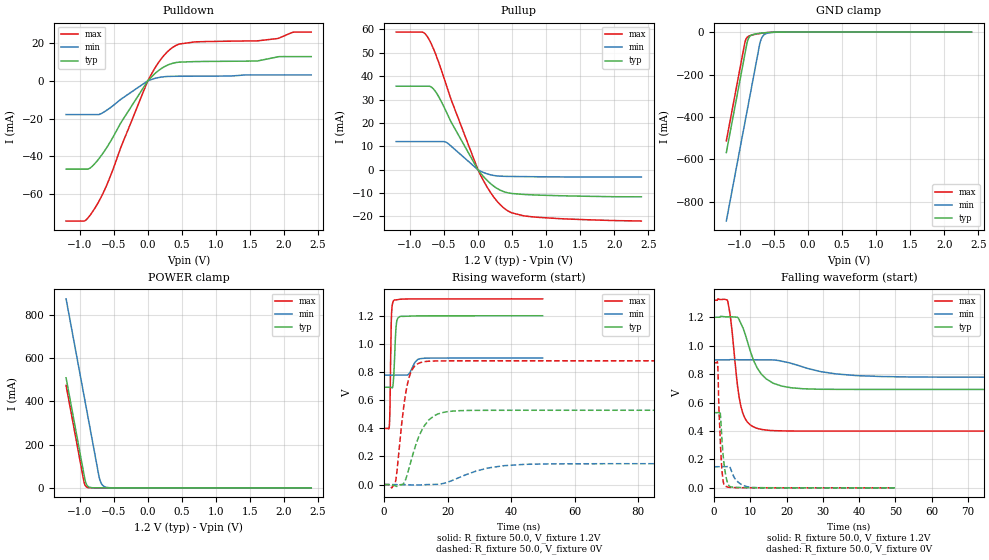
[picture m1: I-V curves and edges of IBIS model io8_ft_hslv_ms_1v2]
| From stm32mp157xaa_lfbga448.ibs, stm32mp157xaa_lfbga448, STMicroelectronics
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[Model]   io8_ft_hslv_ms_1v2
Model_type I/O
Polarity   Non-Inverting
Enable   Active-Low
| CAP_THRESHOLD on pad IOFT is "UDTCAPC" :
| Rising=20.00f vddiom   Falling=80.00f vddiom
| C_comp min and max val. don't necessarily correlate with the min and max pvt
| but are the smallest and greatest pad capacitance found.
| var   typ   min   max
C_comp   3.08865pF  3.06550pF  3.10825pF
|C_comp_pullup   1.81640pF  1.58310pF  1.74795pF
|C_comp_pulldown   1.27225pF  1.48240pF  1.36030pF
Vinl = 360.0mV
Vinh = 792.0mV
Vmeas = 600.0mV   | Reference voltage for timing measurements
Cref  = 50.0pF   | Timing specification test load capacitance value
Rref  = 100.0MOhm   | Timing specification test load resistance value
Vref  = 0V   | Timing specification test load voltage
[Model Spec]
| TIME_THRESHOLD on pin ZIV11 is "CMOS" :
| Rising=40.00f vdd   Falling=60.00f vdd
Vinl 463.60000mV 362.60000mV 506.60000mV
Vinh 741.40000mV 545.40000mV 817.40000mV
| variable   typ   min   max
[Temperature Range] 25.0 140.0 -40.0
| variable   typ   min   max
[Voltage Range] 1.2V 900.0mV 1.32V
| variable   typ   min   max
[POWER Clamp Reference] 1.2V 900.0mV 1.32V
| variable   typ   min   max
[GND Clamp Reference] 0V 0V 0V
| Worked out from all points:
|   slope of the pulldown table from 0 to 0.18 V, typ, clamps not added: 30 ohm
|   slope of the pullup table from 0 to 0.18 V, typ, clamps not added: 31.1 ohm
|   GND clamp passes 1 mA (typ) near -0.52 V on its own axis
|   POWER clamp passes 1 mA (typ) near -0.83 V on its own axis
|   rising waveform, R_fixture 50.0, V_fixture 1.2V: 20-80 % time 608ps typ, 1.71ns min, 359ps max; typ from 0.692 V to 1.2 V
|   falling waveform, R_fixture 50.0, V_fixture 1.2V: 20-80 % time 4.95ns typ, 12.1ns min, 2.49ns max; typ from 1.2 V to 0.692 V
|   rising waveform, R_fixture 50.0, V_fixture 0V: 20-80 % time 5.1ns typ, 11.5ns min, 2.82ns max; typ from 0 V to 0.528 V
|   falling waveform, R_fixture 50.0, V_fixture 0V: 20-80 % time 1.12ns typ, 2.37ns min, 843ps max; typ from 0.528 V to 0 V
[POWER Clamp]
-1.2V     508.8mA    874.1mA    473.5mA
-940mV    66.83mA    432.1mA    31.5mA
-930mV    49.83mA    415.1mA    19.15mA
-910mV    22.88mA    381.1mA    7.077mA
-880mV    7.117mA    330.1mA    1.59mA
-830mV    1.017mA    245.1mA    132uA
-720mV    14.05uA    58.12mA    554nA
-690mV    4.373uA    25.03mA    124.7nA
-650mV    922.4nA    8.136mA    17.22nA
-600mV    132.5nA    1.998mA    1.555nA
-490mV    2.736nA    90.9uA     103pA
2.4V      0A         0A         0A
[GND Clamp]
-1.2V     -567.2mA   -889.7mA   -512.2mA
-930mV    -108.2mA   -430.7mA   -53.23mA
-920mV    -91.21mA   -413.7mA   -40.49mA
-890mV    -43.51mA   -362.7mA   -23.59mA
-860mV    -22.57mA   -311.7mA   -17.89mA
-810mV    -12.11mA   -226.7mA   -13.23mA
-710mV    -6.053mA   -57.05mA   -7.064mA
-680mV    -4.908mA   -27.37mA   -5.632mA
-640mV    -3.605mA   -11.51mA   -3.985mA
-560mV    -1.665mA   -3.218mA   -1.61mA
-360mV    -34.72uA   -209.4uA   -9.248uA
2.4V      3.381nA    1.198uA    162.5pA
| variable   typ   min   max
[Pullup Reference] 1.2V 900.0mV 1.32V
| variable   typ   min   max
[Pulldown Reference] 0V 0V 0V
[Pullup]
-1.2V     35.71mA    12.03mA    58.89mA
-820mV    35.71mA    12.03mA    58.89mA
-730mV    35.71mA    12.03mA    56.33mA
-620mV    33.3mA     12.03mA    49.33mA
-460mV    24.5mA     11.63mA    35.82mA
-400mV    20.74mA    10.25mA    30.47mA
0V        5.9pA      1.254nA    2.839pA
200mV     -6.284mA   -2.265mA   -10.37mA
390mV     -9.473mA   -2.816mA   -16.58mA
500mV     -10.16mA   -2.878mA   -18.47mA
810mV     -10.76mA   -2.985mA   -20.17mA
2.4V      -11.58mA   -3.134mA   -21.93mA
[Pulldown]
-1.2V     -46.7mA    -17.86mA   -74.13mA
-930mV    -46.7mA    -17.86mA   -74.13mA
-770mV    -43.45mA   -17.86mA   -66.94mA
-580mV    -33.98mA   -14.99mA   -53.18mA
0V        0A         -3pA       0A
170mV     5.742mA    1.791mA    10.3mA
340mV     8.972mA    2.348mA    16.97mA
690mV     10.15mA    2.431mA    20.56mA
1.61V     10.49mA    3.108mA    21.11mA
1.91V     12.66mA    3.108mA    22.36mA
2.14V     12.8mA     3.108mA    25.73mA
2.4V      12.8mA     3.108mA    25.78mA
[Ramp]
dV/dt_r 316.9919mV/5.10359ns 89.06671mV/11.51485ns 527.8372mV/2.82332ns
dV/dt_f 304.66124mV/4.94572ns 73.1992mV/12.07723ns 552.41113mV/2.48796ns
R_load = 50.0
| Removed startup time: 0s 0s 0s  .
| Removed end time: 49.9ns.
[Rising Waveform]
R_fixture   = 50.0
V_fixture   = 1.2V
V_fixture_min = 900.0mV
V_fixture_max = 1.32V
0s        692.2mV    778mV      399.3mV
1.7ns     692.5mV    778.1mV    417.6mV
1.9ns     692.5mV    778.1mV    547.9mV
2.2ns     691.9mV    778.1mV    1.042V
2.4ns     690.5mV    778.1mV    1.22V
3.2ns     823.1mV    778.1mV    1.311V
3.9ns     1.141V     778.1mV    1.313V
5ns       1.194V     778.1mV    1.317V
11.7ns    1.199V     895.9mV    1.32V
49.9ns    1.2V       900mV      1.32V
| Removed startup time: 0s 0s 0s  .
| Removed end time: 299.9ns.
[Falling Waveform]
R_fixture   = 50.0
V_fixture   = 1.2V
V_fixture_min = 900.0mV
V_fixture_max = 1.32V
0s        1.2V       900mV      1.32V
3.8ns     1.203V     899.7mV    1.31V
4.7ns     1.203V     902.5mV    1.163V
6.8ns     1.189V     901mV      655mV
8.1ns     1.117V     900.8mV    513.6mV
10.9ns    895.9mV    900.9mV    428.6mV
14.2ns    770.8mV    900.6mV    406.9mV
21.3ns    703.7mV    875.8mV    399.7mV
46.4ns    692.2mV    782.9mV    399.3mV
299.9ns   692.2mV    778mV      399.3mV
| Removed startup time: 0s 0s 0s  .
| Removed end time: 299.9ns.
[Rising Waveform]
R_fixture   = 50.0
V_fixture   = 0V
V_fixture_min = 0V
V_fixture_max = 0V
0s        25.9nV     725nV      -2.471uV
3.6ns     -8.736mV   -3.709uV   16.33mV
6.3ns     11.17mV    80.74uV    568mV
8.1ns     134.4mV    -2.378mV   775.5mV
10.9ns    338.9mV    -3.138mV   861.6mV
13.1ns    430.1mV    -398.1uV   874.8mV
19.8ns    517.9mV    15.05mV    879.5mV
32.7ns    528mV      117.5mV    879.7mV
44.3ns    528.2mV    143.8mV    879.7mV
299.9ns   528.3mV    148.4mV    879.7mV
| Removed startup time: 0s 0s 0s  .
| Removed end time: 49.9ns.
[Falling Waveform]
R_fixture   = 50.0
V_fixture   = 0V
V_fixture_min = 0V
V_fixture_max = 0V
0s        528.3mV    148.5mV    879.7mV
1ns       528.4mV    148.5mV    877.6mV
1.3ns     528mV      148.5mV    589.7mV
1.7ns     531.1mV    148.5mV    340.5mV
2ns       409.7mV    148.5mV    187.9mV
2.5ns     227.8mV    148.5mV    47.74mV
3ns       120.1mV    148.4mV    13.46mV
4.3ns     10.34mV    149.4mV    3.566mV
10.1ns    815.9uV    4.118mV    208.1uV
49.9ns    106.3nV    17.68uV    -47.36nV
